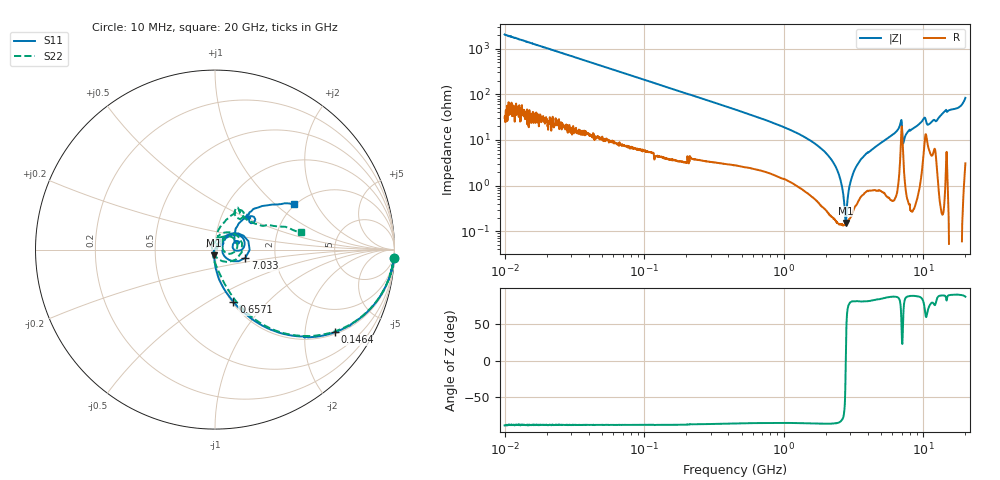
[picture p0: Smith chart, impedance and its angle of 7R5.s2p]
!Keysight Technologies,P5008B,MY61100088,A.16.20.02
!Date: Monday, November 06, 2023 16:09:04
!Correction: S11(C  2-Port  )
!S21(C  2-Port  )
!S12(C  2-Port  )
!S22(C  2-Port  )
!S2P File: Measurements: S11, S21, S12, S22:Log Frequency Sweep
# Hz S  dB  R 50
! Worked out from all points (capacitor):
!   1601 points, 10 MHz to 20 GHz, reference 50 ohm
!   read as one part in series: C = 7.81 pF near 10.39 MHz
!   lowest |Z| = 152 mohm at 2.772 GHz (marker M1)
!   series resonance near 2.779 GHz, so ESL is about 420 pH
!   S11 on the Smith chart (normalised r, x): 10 MHz: 1, -41; 146.4 MHz: 1.06, -2.85; 657.1 MHz: 1.02, -0.65; 7.033 GHz: 1.40, -0.13; 20 GHz: 1.98, +1.34
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1e7  -0.02 -2.8  -26.21 86.3  -26.21 86.4  -0.01 -2.8
3.555162e7  -0.16 -9.7  -15.49 78.8  -15.49 78.8  -0.16 -9.8
1.263918e8  -1.44 -30.9  -5.81 57.6  -5.84 57.4  -1.49 -31.0
1.464456e8  -1.83 -34.7  -4.92 53.8  -4.96 53.5  -1.89 -34.7
4.472136e8  -7.43 -62.8  -1.08 24.0  -1.07 24.0  -7.83 -62.7
6.570972e8  -10.21 -70.6  -0.62 16.5  -0.61 16.5  -10.94 -69.3
1.589917e9  -18.81 -87.0  -0.15 4.4  -0.15 4.4  -20.24 -84.7
2.771802e9  -29.64 -102.1  -0.09 -2.0  -0.10 -2.0  -28.17 -105.6
3.106545e9  -35.08 -118.7  -0.11 -3.2  -0.11 -3.3  -30.13 -105.7
3.53169e9  -50.94 112.6  -0.11 -4.6  -0.12 -4.6  -33.94 -104.6
3.846973e9  -39.86 61.9  -0.10 -5.5  -0.11 -5.6  -38.45 -92.8
4.352721e9  -39.79 47.2  -0.07 -7.1  -0.08 -7.1  -41.71 -22.2
5.652411e9  -31.38 64.1  -0.04 -11.3  -0.05 -11.3  -29.49 68.0
6.802936e9  -18.89 47.8  -0.33 -18.0  -0.33 -18.0  -19.57 62.9
7.032964e9  -15.14 -15.0  -1.42 -11.1  -1.42 -11.2  -17.78 -25.7
7.445538e9  -27.77 2.3  -0.08 -13.8  -0.08 -13.8  -32.53 137.7
8.344716e9  -26.86 43.5  -0.02 -18.0  -0.02 -18.0  -28.11 92.7
1.009107e10  -16.77 34.5  -0.56 -26.6  -0.57 -26.6  -18.56 35.5
1.11497e10  -20.03 8.7  -0.44 -23.4  -0.45 -23.4  -27.28 31.1
1.400536e10  -12.60 46.9  -0.20 -33.6  -0.20 -33.6  -12.80 61.8
1.801527e10  -11.63 47.1  -0.34 -48.9  -0.34 -48.9  -12.13 39.6
2e10  -5.88 29.7  -1.63 -66.4  -1.63 -66.4  -6.21 11.2
